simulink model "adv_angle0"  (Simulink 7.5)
settings: Solver=ode113  StartTime=0.0  StopTime=2  MaxStep=1e-4  MinStep=1e-5  RelTol=1e-5
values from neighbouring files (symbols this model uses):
  B = 0.0001    [adv1.m]    (also in adv1_plot_eaia.m; adv1_plot_te_speed.m; lookup01_plot.m; NEW_VAR .m)
  BV = 24    [adv1.m]    (also in adv1_plot_eaia.m; adv1_plot_te_speed.m; lookup01_plot.m; NEW_VAR .m)
  J = .0001    (= 0.0001)    [adv1.m]    (also in adv1_plot_eaia.m; adv1_plot_te_speed.m; lookup01_plot.m; NEW_VAR .m)
  kw = 0.0445    [adv1.m]    (also in adv1_plot_eaia.m; adv1_plot_te_speed.m; lookup01_plot.m = 0.0365; NEW_VAR .m)
  L = .00192    (= 0.00192)    [adv1.m]    (also in adv1_plot_eaia.m; adv1_plot_te_speed.m; lookup01_plot.m; NEW_VAR .m)
  P = 4    [adv1.m]    (also in adv1_plot_eaia.m; adv1_plot_te_speed.m; lookup01_plot.m; NEW_VAR .m)
  R = 1.5    [adv1.m]    (also in adv1_plot_eaia.m; adv1_plot_te_speed.m; lookup01_plot.m; NEW_VAR .m)
  T0 = 0.0001    [adv1.m]    (also in adv1_plot_eaia.m; adv1_plot_te_speed.m; lookup01_plot.m; NEW_VAR .m)
  W0 = 2    [adv1.m]    (also in adv1_plot_eaia.m; adv1_plot_te_speed.m; lookup01_plot.m; NEW_VAR .m)

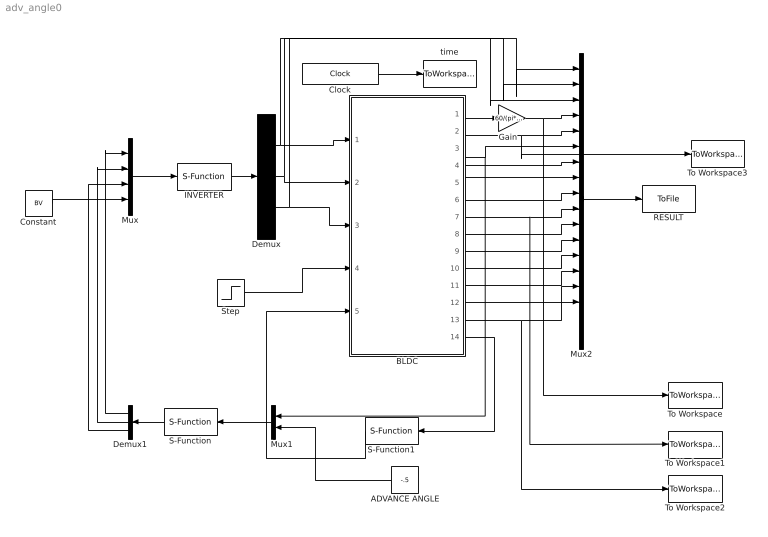
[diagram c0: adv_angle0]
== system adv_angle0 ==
  ADVANCE ANGLE : Constant  Value=-.5  OutDataType=fixdt(1, 16)  OutScaling=2^0
  BLDC : Subsystem
  Clock : Clock
  Constant : Constant  Value=BV  OutDataType=fixdt(1, 16)  OutScaling=2^0
  Demux : Demux  Outputs=3
  Demux1 : Demux  Outputs=3
  Gain : Gain  Gain=60/(pi*P)  ParameterDataType=fixdt(1, 16)  ParameterScaling=2^0  OutDataType=fixdt(1, 16)  OutScaling=2^0
  INVERTER : S-Function  FunctionName=inverter  Parameters=vmax  EnableBusSupport=off  mask{vmax=50}
      mask prompts: vmax "maximum dc bus"
  Mux : Mux
  Mux1 : Mux  Inputs=2
  Mux2 : Mux  Inputs=18
  RESULT : ToFile  Filename=bldc_advangle
  S-Function : S-Function  FunctionName=BLDC_adv_2in  Parameters=angle  EnableBusSupport=off  mask{angle=0}
      mask prompts: angle "advance  angle"
  S-Function1 : S-Function  FunctionName=sam_adv_ktc  Parameters=R,L,J,P,kw  EnableBusSupport=off
  Step : Step  After=0.4  SampleTime=0
  To Workspace : ToWorkspace  VariableName=speed1  SampleTime=-1  SaveFormat=Array
  To Workspace1 : ToWorkspace  VariableName=ea1  SampleTime=-1  SaveFormat=Array
  To Workspace2 : ToWorkspace  VariableName=ia1  SampleTime=-1  SaveFormat=Array
  To Workspace3 : ToWorkspace  VariableName=te1  SampleTime=-1  SaveFormat=Array
  time : ToWorkspace  VariableName=time  SampleTime=-1  SaveFormat=Array
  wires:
  INVERTER/1 -> Demux/1
  Mux/1 -> INVERTER/1
  BLDC/1(W) -> Gain/1
  Clock/1 -> time/1
  S-Function/1 -> Demux1/1
  Constant/1 -> Mux/4
  BLDC/14(outadv) -> S-Function1/1
  Mux1/1 -> S-Function/1
  BLDC/3(Phi) -> Mux1/1, Mux2/6
  S-Function1/1 -> BLDC/5(inadv)
  Demux/1 -> BLDC/1(Va), Mux2/1
  Demux/2 -> BLDC/2(Vb), Mux2/2
  Demux/3 -> BLDC/3(Vc), Mux2/3
  Demux1/1 -> Mux/1
  Demux1/2 -> Mux/2
  Demux1/3 -> Mux/3
  ADVANCE ANGLE/1 -> Mux1/2
  Gain/1 -> Mux2/4, To Workspace/1
  BLDC/2(Te) -> Mux2/5, To Workspace3/1
  BLDC/4(HA) -> Mux2/7
  BLDC/5(HB) -> Mux2/8
  BLDC/6(HC) -> Mux2/9
  BLDC/7(ea) -> Mux2/10, To Workspace1/1
  BLDC/8(eb) -> Mux2/11
  BLDC/9(ec) -> Mux2/12
  BLDC/10(theta) -> Mux2/13
  BLDC/11(ic) -> Mux2/14
  BLDC/12(ib) -> Mux2/15
  BLDC/13(ia) -> Mux2/16, To Workspace2/1
  Mux2/1 -> RESULT/1
  Step/1 -> BLDC/4(Tload)

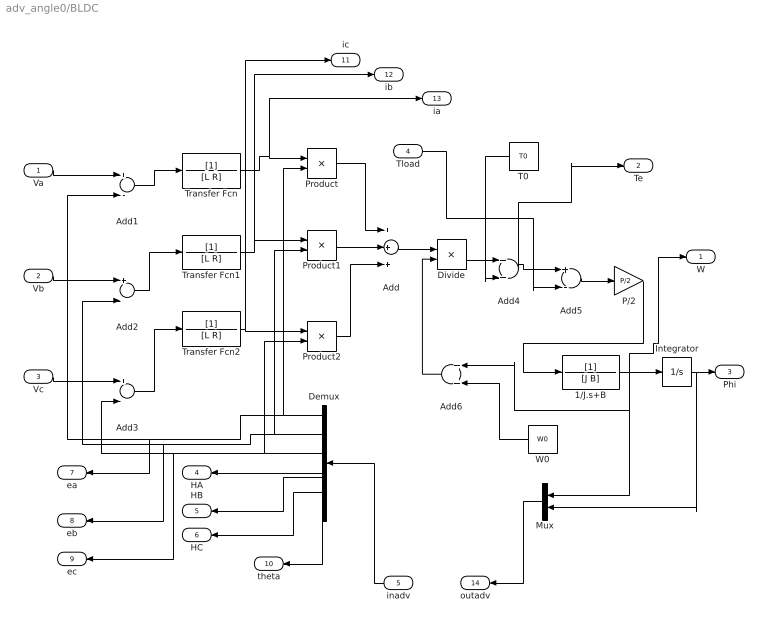
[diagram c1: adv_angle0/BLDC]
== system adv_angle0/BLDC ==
  Va : Inport  OutDataType=fixdt(1, 16)  OutScaling=2^0
  Vb : Inport  Port=2  OutDataType=fixdt(1, 16)  OutScaling=2^0
  Vc : Inport  Port=3  OutDataType=fixdt(1, 16)  OutScaling=2^0
  Tload : Inport  Port=4  OutDataType=fixdt(1, 16)  OutScaling=2^0
  inadv : Inport  Port=5  OutDataType=fixdt(1, 16)  OutScaling=2^0
  1/J.s+B : TransferFcn  Denominator=[J B]
  Add : Sum  Inputs=+++  OutDataType=fixdt(1, 16)  OutScaling=2^-10
  Add{1..3,5} (4 alike) : Sum  Inputs=+-  OutDataType=fixdt(1, 16)  OutScaling=2^-10
  Add4 : Sum  OutDataType=fixdt(1, 16)  OutScaling=2^-10
  Add6 : Sum  OutDataType=fixdt(1, 16)  OutScaling=2^-10
  Demux : Demux  Outputs=7
  Divide : Product  Inputs=*/  OutDataType=fixdt(1, 16)  OutScaling=2^-10
  Integrator : Integrator
  Mux : Mux  Inputs=2
  P/2 : Gain  Gain=P/2  ParameterDataType=fixdt(1, 16)  ParameterScaling=2^0  OutDataType=fixdt(1, 16)  OutScaling=2^0
  Product : Product  OutDataType=fixdt(1, 16)  OutScaling=2^0
  Product1 : Product  OutDataType=fixdt(1, 16)  OutScaling=2^0
  Product2 : Product  OutDataType=fixdt(1, 16)  OutScaling=2^0
  T0 : Constant  Value=T0  OutDataType=fixdt(1, 16)  OutScaling=2^0
  Transfer Fcn : TransferFcn  Denominator=[L R]
  Transfer Fcn1 : TransferFcn  Denominator=[L R]
  Transfer Fcn2 : TransferFcn  Denominator=[L R]
  W0 : Constant  Value=W0  OutDataType=fixdt(1, 16)  OutScaling=2^0
  W : Outport  OutDataType=fixdt(1, 16)  OutScaling=2^0
  Te : Outport  Port=2  OutDataType=fixdt(1, 16)  OutScaling=2^0
  Phi : Outport  Port=3  OutDataType=fixdt(1, 16)  OutScaling=2^0
  HA : Outport  Port=4  OutDataType=fixdt(1, 16)  OutScaling=2^0
  HB : Outport  Port=5  OutDataType=fixdt(1, 16)  OutScaling=2^0
  HC : Outport  Port=6  OutDataType=fixdt(1, 16)  OutScaling=2^0
  ea : Outport  Port=7  OutDataType=fixdt(1, 16)  OutScaling=2^0
  eb : Outport  Port=8  OutDataType=fixdt(1, 16)  OutScaling=2^0
  ec : Outport  Port=9  OutDataType=fixdt(1, 16)  OutScaling=2^0
  theta : Outport  Port=10  OutDataType=fixdt(1, 16)  OutScaling=2^0
  ic : Outport  Port=11  OutDataType=fixdt(1, 16)  OutScaling=2^0
  ib : Outport  Port=12  OutDataType=fixdt(1, 16)  OutScaling=2^0
  ia : Outport  Port=13  OutDataType=fixdt(1, 16)  OutScaling=2^0
  outadv : Outport  Port=14  OutDataType=fixdt(1, 16)  OutScaling=2^0
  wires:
  Add1/1 -> Transfer Fcn/1
  Add2/1 -> Transfer Fcn1/1
  Add3/1 -> Transfer Fcn2/1
  Transfer Fcn/1 -> Product/1, ia/1
  Transfer Fcn1/1 -> Product1/1, ib/1
  Transfer Fcn2/1 -> Product2/1, ic/1
  Demux/1 -> Add1/2, ea/1, Product/2
  Demux/2 -> Product1/2, Add2/2, eb/1
  Va/1 -> Add1/1
  Vb/1 -> Add2/1
  Vc/1 -> Add3/1
  Demux/3 -> Product2/2, Add3/2, ec/1
  Product/1 -> Add/1
  Product1/1 -> Add/2
  Product2/1 -> Add/3
  Add/1 -> Divide/1
  Add5/1 -> P/2/1
  Divide/1 -> Add4/1
  T0/1 -> Add4/2
  Add4/1 -> Add5/1, Te/1
  Tload/1 -> Add5/2
  P/2/1 -> 1/J.s+B/1
  1/J.s+B/1 -> Integrator/1, W/1, Add6/1, Mux/1
  Add6/1 -> Divide/2
  W0/1 -> Add6/2
  Integrator/1 -> Phi/1, Mux/2
  Demux/4 -> HA/1
  Demux/5 -> HB/1
  Demux/6 -> HC/1
  Demux/7 -> theta/1
  inadv/1 -> Demux/1
  Mux/1 -> outadv/1
